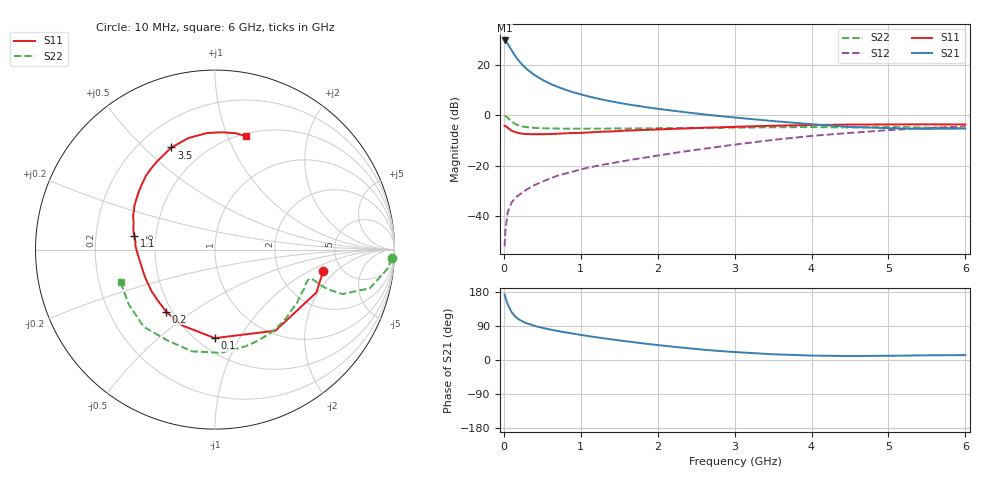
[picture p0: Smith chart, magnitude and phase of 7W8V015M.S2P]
! Infineon Technologies  Discrete & RF Semiconductors
! BFS17W
! Si NPN RF Bipolar Junction Transistor in SOT323
! VCE = 8 V  IC = 15 mA
! Common Emitter S-Parameters:  August  1999
# GHz  S  MA  R  50
!  f  S11  S21  S12  S22
! GHz  MAG  ANG  MAG  ANG  MAG  ANG  MAG  ANG
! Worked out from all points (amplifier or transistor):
!   36 points, 10 MHz to 6 GHz, reference 50 ohm
!   highest |S21| = 29.7 dB at 10 MHz (marker M1)
!   |S21| within 3 dB of that: start of sweep to 82.8 MHz
!   unconditionally stable (mu >= 1): 367.1 MHz to 2.088 GHz; 5.544 GHz to end of sweep
!   at 250 MHz: K = 0.88, MSG = 25.1 dB, |S12| = -30.5 dB
!   at 1.4 GHz: K = 1.15, MAG = 9.9 dB, |S12| = -19.1 dB
!   at 6 GHz: K = 1.03, MAG = -1.5 dB, |S12| = -4.5 dB
!   S11 on the Smith chart (normalised r, x): 10 MHz: 3.61, -1.39; 100 MHz: 0.61, -0.79; 200 MHz: 0.46, -0.40; 1.1 GHz: 0.38, +0.07; 3.5 GHz: 0.33, +0.61; 6 GHz: 0.53, +1.17
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0.01  0.6143 -11.3  30.57 172.8  0.0025 84.4  0.9866 -2.8
0.02  0.6134 -22.9  30.01 165.5  0.0049 84.3  0.9649 -6.5
0.05  0.5635 -53.3  26.32 147.1  0.0117 68.7  0.8896 -14.0
0.1  0.4932 -90.1  19.53 126.7  0.0183 60.2  0.7531 -19.2
0.15  0.4606 -113.6  14.86 114.3  0.023 57.8  0.6675 -19.4
0.2  0.4401 -128.2  11.8 106.6  0.0262 59.7  0.622 -18.6
0.25  0.4263 -138.7  9.69 101.0  0.0297 59.2  0.5942 -17.7
0.3  0.4229 -146.6  8.204 96.7  0.0337 61.4  0.5787 -17.2
0.4  0.4188 -157.7  6.267 90.0  0.0409 64.2  0.5591 -16.8
0.5  0.419 -165.0  5.061 84.9  0.0479 65.9  0.5515 -17.0
0.6  0.4223 -170.5  4.227 80.5  0.055 67.3  0.5468 -17.8
0.7  0.4288 -174.9  3.655 76.6  0.063 68.5  0.5434 -19.0
0.9  0.4439 177.4  2.865 69.6  0.0758 69.7  0.5398 -22.0
1.1  0.4547 170.6  2.365 63.0  0.0911 70.5  0.5406 -25.7
1.3  0.472 164.7  2.017 57.2  0.1047 71.1  0.5405 -29.9
1.6  0.496 156.8  1.653 49.1  0.1258 72.4  0.5435 -36.3
2.2  0.5346 142.3  1.226 35.0  0.1761 73.7  0.5544 -51.0
2.8  0.5749 128.3  0.964 23.8  0.2373 72.5  0.5616 -67.0
3.5  0.6186 113.1  0.765 15.1  0.3235 67.9  0.5762 -86.7
4.5  0.651 94.0  0.585 10.4  0.4443 55.9  0.5711 -118.1
5.5  0.6585 80.1  0.535 12.3  0.5543 42.7  0.5694 -147.8
6  0.6549 74.6  0.542 12.9  0.5987 36.1  0.5558 -161.1
